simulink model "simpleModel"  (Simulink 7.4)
settings: Solver=ode45  StartTime=0.0  StopTime=800  RelTol=1e-3
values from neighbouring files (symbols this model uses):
  eta = 2    [project4_solution.m]
  I_0 = 1    [project4_solution.m]
  N = 400    [project4_solution.m]
  Omega = power(2, 14)    [project4_solution.m]

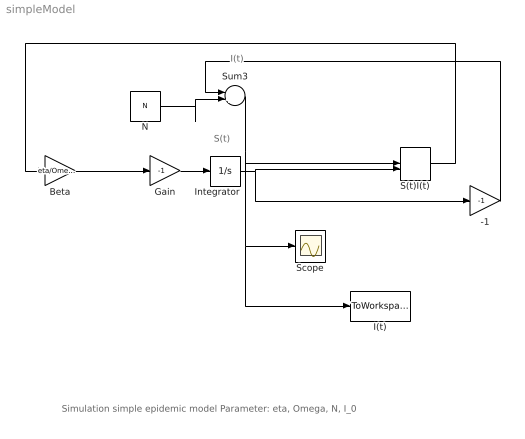
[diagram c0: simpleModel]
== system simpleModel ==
  note: S(t)
  note: I(t)
  note: Simulation simple epidemic model Parameter: eta, Omega, N, I_0
  -1 : Gain  Gain=-1
  Beta : Gain  Gain=eta/Omega
  Gain : Gain  Gain=-1
  I(t) : ToWorkspace  VariableName=I_t  SampleTime=1  SaveFormat=Array
  Integrator : Integrator  InitialCondition=N-I_0
  N : Constant  Value=N  VectorParams1D=off
  S(t)I(t) : DotProduct  OutDataType=sfix(16)  OutScaling=2^-10
  Scope : Scope
  Sum3 : Sum  Inputs=|++
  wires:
  Integrator/1 -> -1/1, S(t)I(t)/2
  Gain/1 -> Integrator/1
  Beta/1 -> Gain/1
  Sum3/1 -> I(t)/1, Scope/1, S(t)I(t)/1
  S(t)I(t)/1 -> Beta/1
  -1/1 -> Sum3/1
  N/1 -> Sum3/2
